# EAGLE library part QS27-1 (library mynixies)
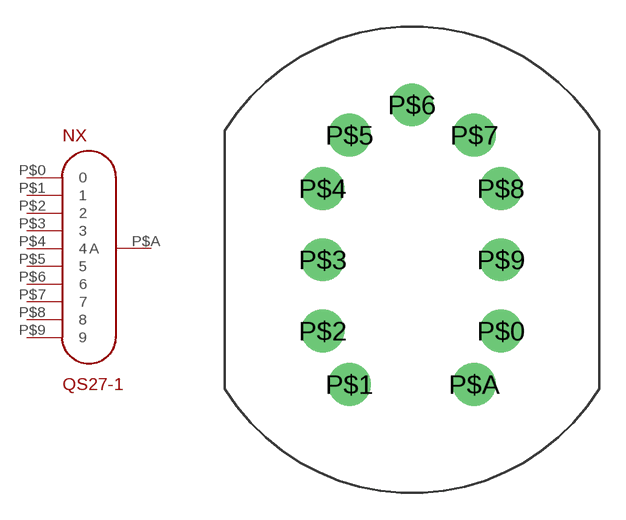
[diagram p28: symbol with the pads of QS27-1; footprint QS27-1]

Designator prefix NX

## QS27-1DSUB  [QS27-1]
P$0  0  pas
P$1  1  pas
P$2  2  pas
P$3  3  pas
P$4  4  pas
P$5  5  pas
P$6  6  pas
P$7  7  pas
P$8  8  pas
P$9  9  pas
P$A  A  pas

## Footprint QS27-1 (pad centres in mm)
drill 1.6: P$0 5,-4; P$1 -3.5,-7; P$2 -5,-4; P$3 -5,0; P$4 -5,4; P$5 -3.5,7; P$6 0,8.7; P$7 3.5,7; P$8 5,4; P$9 5,0; P$A 3.5,-7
